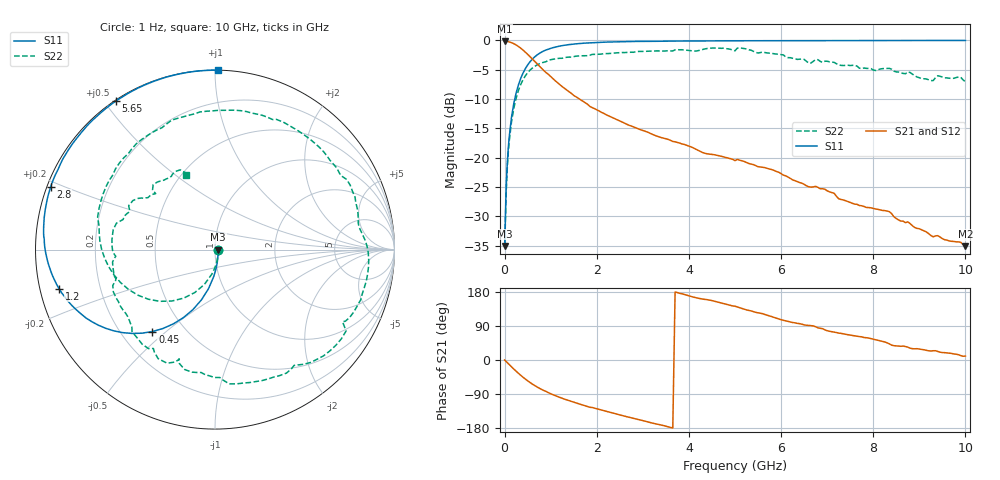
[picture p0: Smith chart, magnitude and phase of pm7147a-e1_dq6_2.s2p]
# GHz S DB R 50
! S-Parameters data
! Freq  dbS11  angS11  dbS21  angS21  dbS12  angS12  dbS22  angS22
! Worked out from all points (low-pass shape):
!   279 points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, 1 Hz to 10 GHz, reference 50 ohm
!   highest |S21| = -0.16 dB at 158.5 Hz (marker M1); lowest = -35.1 dB at 10 GHz (marker M2)
!   |S21| within 3 dB of the highest: start of sweep to 601.8 MHz
!   lowest |S11| = -35.0 dB at 2.5 Hz (marker M3), VSWR 1.04, Z = 51.8 - j3.44e-07 ohm
!   |S11| at or under -10 dB: start of sweep to 220.7 MHz
!   |S22| runs from -35.0 to -1.3 dB; largest |S21 - S12| = 0
!   S11 on the Smith chart (normalised r, x): 1 Hz: 1.04, -0.00; 450 MHz: 0.33, -0.45; 1.2 GHz: 0.06, -0.12; 2.8 GHz: 0.01, +0.18; 5.65 GHz: 0.00, +0.54; 10 GHz: 0.00, +1.02
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1e-09  -35.04 -0.0  -0.16 -0.0  -0.16 -0.0  -35.04 -0.0
2.5e-09  -35.04 -0.0  -0.16 -0.0  -0.16 -0.0  -35.04 -0.0
1.585e-07  -35.04 -0.0  -0.16 -0.0  -0.16 -0.0  -35.04 -0.0
0.03162278  -25.87 -72.3  -0.17 -3.9  -0.17 -3.9  -26.52 -72.2
0.06309573  -20.32 -85.2  -0.20 -7.7  -0.20 -7.7  -21.05 -87.5
0.15  -13.08 -99.5  -0.38 -18.1  -0.38 -18.1  -13.86 -106.9
0.45  -4.81 -127.4  -1.99 -50.4  -1.99 -50.4  -6.04 -149.4
0.75  -2.23 -146.9  -4.33 -74.2  -4.33 -74.2  -4.00 -180.0
1.2  -0.95 -166.0  -7.54 -98.8  -7.54 -98.8  -3.04 146.8
1.7  -0.48 -180.0  -10.39 -118.9  -10.39 -118.9  -2.61 118.4
2.2  -0.28 169.5  -12.66 -135.4  -12.66 -135.4  -2.24 93.4
2.8  -0.17 159.1  -14.76 -153.9  -14.76 -153.9  -2.02 66.1
3.35  -0.14 151.0  -16.45 -170.3  -16.45 -170.3  -1.78 42.1
4.4  -0.08 137.4  -19.34 159.1  -19.34 159.1  -1.37 -1.2
5.05  -0.06 129.9  -20.29 140.1  -20.29 140.1  -1.31 -31.8
5.65  -0.04 123.6  -21.70 120.0  -21.70 120.0  -2.06 -62.9
6.05  -0.04 119.7  -22.97 104.8  -22.97 104.8  -2.47 -83.9
6.7  -0.03 113.6  -24.98 89.9  -24.98 89.9  -3.55 -109.5
7.6  -0.01 106.0  -27.92 64.0  -27.92 64.0  -4.25 -157.5
8.35  -0.01 100.2  -29.21 42.6  -29.21 42.6  -4.77 168.8
8.85  -0.01 96.6  -31.61 29.9  -31.61 29.9  -5.75 146.5
10  -0.00 89.1  -35.09 10.4  -35.09 10.4  -7.04 111.2
